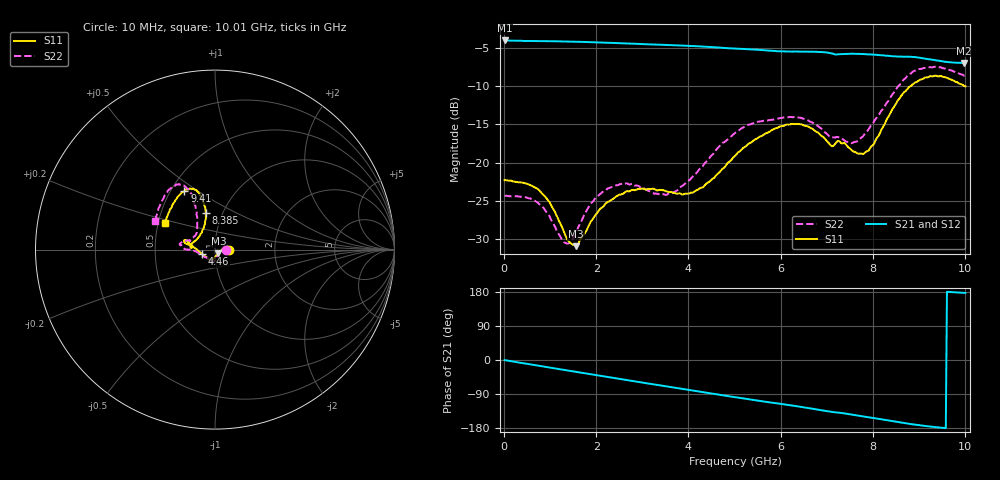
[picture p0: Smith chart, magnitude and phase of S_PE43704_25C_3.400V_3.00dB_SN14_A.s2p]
! Device ID: PE43704
! Dir: z:\PE43704\PE43704_Char_1_20130516\PE43704\AMB\3p400V\3p00dB
! Serial: 14
! Insertion: A
! Impedance: 50 ohm
! Temp: Amb
! VDD: 3.400V
! Attenuation Step: 3.00dB
! IDD: 1.141048e-01mA
#  Hz  S  RI  R  50
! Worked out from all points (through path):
!   401 points, 10 MHz to 10.01 GHz, reference 50 ohm
!   highest |S21| = -4.01 dB at 10 MHz (marker M1); lowest = -7.0 dB at 9.985 GHz (marker M2)
!   group delay of S21, straight-line fit = 52.1 ps
!   lowest |S11| = -30.9 dB at 1.56 GHz (marker M3), VSWR 1.06, Z = 51.9 - j2.22 ohm
!   |S11| at or under -10 dB: start of sweep to 8.816 GHz; 9.998286 GHz to end of sweep
!   |S22| runs from -30.6 to -7.5 dB; largest |S21 - S12| = 0.0039
!   S11 on the Smith chart (normalised r, x): 10 MHz: 1.17, +0.00; 4.46 GHz: 0.87, -0.05; 8.385 GHz: 0.83, +0.36; 9.41 GHz: 0.59, +0.44; 10.01 GHz: 0.54, +0.18
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1e7  0.0768 0.000211  0.6303 -0.0026  0.6305 -0.00251  0.0606 0.000247
7.6e8  0.0632 0.0187  0.6019 -0.1655  0.602 -0.1653  0.051 0.0168
1.31e9  0.0341 -0.00527  0.5559 -0.2757  0.556 -0.2757  0.0278 -0.0113
1.56e9  0.0187 -0.0214  0.528 -0.3218  0.5279 -0.3218  0.0166 -0.0306
1.685e9  0.0117 -0.0304  0.5122 -0.344  0.5122 -0.3439  0.0106 -0.0405
1.985e9  -0.00261 -0.0455  0.4704 -0.3924  0.4706 -0.3923  0.000634 -0.059
2.385e9  -0.0155 -0.0564  0.4085 -0.4487  0.4087 -0.4486  -0.0108 -0.0696
3.36e9  -0.0264 -0.0608  0.2358 -0.5425  0.2364 -0.5422  -0.0251 -0.0567
3.735e9  -0.0352 -0.0518  0.1641 -0.5627  0.1649 -0.5626  -0.0469 -0.0455
4.46e9  -0.0708 -0.026  0.0218 -0.572  0.0222 -0.5725  -0.1073 -0.0098
5.01e9  -0.1104 0.00757  -0.0784 -0.5524  -0.0782 -0.5526  -0.1563 0.00011
5.985e9  -0.164 0.0532  -0.2308 -0.4837  -0.2283 -0.484  -0.1942 0.0251
6.685e9  -0.1635 0.0343  -0.3313 -0.4158  -0.3319 -0.4154  -0.1777 0.0445
7.485e9  -0.1169 0.0447  -0.4113 -0.3113  -0.4114 -0.3114  -0.1132 0.0762
7.76e9  -0.0895 0.0716  -0.4371 -0.2695  -0.4368 -0.2705  -0.1009 0.1061
7.985e9  -0.07 0.1084  -0.4527 -0.2344  -0.4524 -0.2364  -0.0992 0.1479
8.36e9  -0.0511 0.1985  -0.4684 -0.172  -0.4675 -0.1739  -0.1079 0.237
8.385e9  -0.0506 0.2062  -0.4694 -0.167  -0.4675 -0.1694  -0.109 0.2447
8.86e9  -0.0886 0.3123  -0.484 -0.0886  -0.4808 -0.0895  -0.168 0.3536
9.41e9  -0.1702 0.3256  -0.4654 -0.0175  -0.4652 -0.0166  -0.2465 0.3412
9.985e9  -0.2727 0.1614  -0.4479 0.0224  -0.4491 0.0235  -0.3286 0.1685
1.001e10  -0.2774 0.1505  -0.4493 0.0234  -0.4518 0.0237  -0.3318 0.1595
